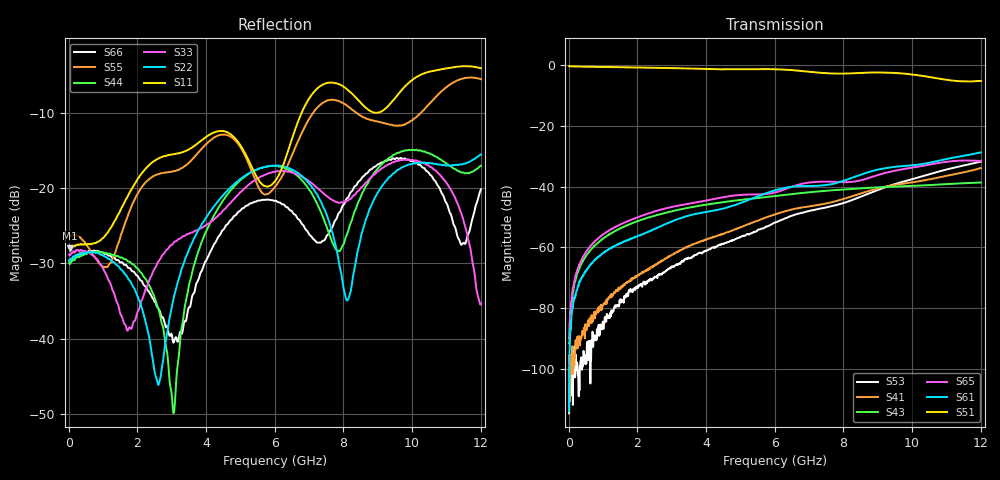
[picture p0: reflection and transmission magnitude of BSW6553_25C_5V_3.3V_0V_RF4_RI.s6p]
! Agilent Technologies	N5230C	MY49001333	A.09.33.09
!	Test time	=	2026-05-26
!	Product	=	BSW6553
!	Temp	=	25C
!	Logic	=	RF4
!	Port1	=	RFC
!	Port2	=	RF1
!	Port3	=	RF2
!	Port4	=	RF3
!	Port5	=	RF4
!	Port6	=	RF5
!S6P File: Measurements: <S11,S12,S13,S14,S15,S16>,
!<S21,S22,S23,S24,S25,S26>,
!<S31,S32,S33,S34,S35,S36>,
!<S41,S42,S43,S44,S45,S46>,
!<S51,S52,S53,S54,S55,S56>,
!<S61,S62,S63,S64,S65,S66>;
# HZ S RI R 50
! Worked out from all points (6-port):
!   1201 points, 10 MHz to 12.01 GHz, reference 50 ohm
!   strongest paths, dB at 10 MHz, 3.01 GHz, 6.01 GHz, 9.01 GHz, 12.01 GHz:
!     S51: -0.5, -1.2, -1.5, -2.6, -5.3
!     S61: -113.8, -51.5, -41.2, -34.5, -28.8
!     S65: -89.7, -46.7, -42.0, -36.2, -31.6
!     S43: -91.4, -48.1, -43.1, -40.3, -38.7
!     S41: -97.4, -62.4, -49.1, -40.6, -33.9
!     S53: -114.4, -66.5, -51.8, -41.1, -31.8
!   lowest |S11| = -28.0 dB at 40 MHz (marker M1), VSWR 1.08, Z = 54.1 - j0.492 ohm
!   |S11| at or under -10 dB: start of sweep to 6.782 GHz
